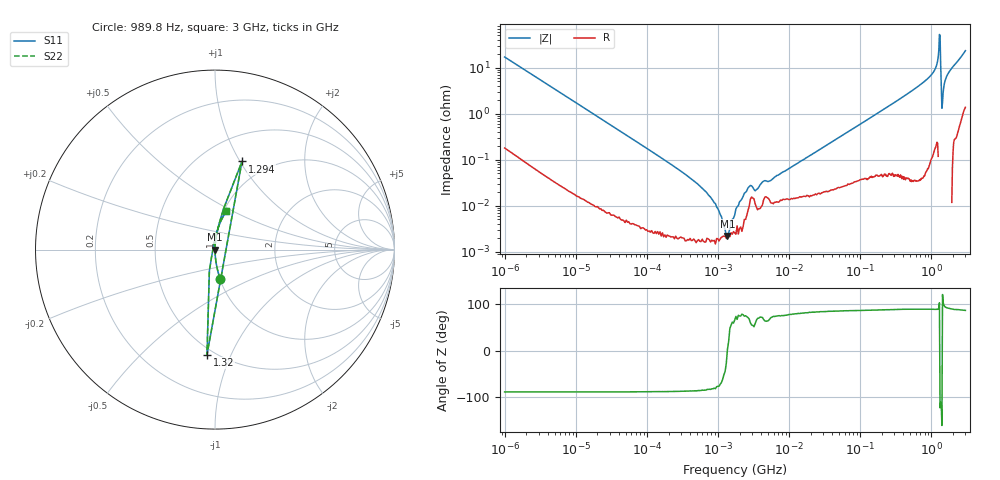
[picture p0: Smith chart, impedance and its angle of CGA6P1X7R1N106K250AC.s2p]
! S-Parameter Data Generated by TDK Corporation
! Copyright(C) 2020 TDK Corporation.
! All Rights Reserved.
! TDK P/N: CGA6P1X7R1N106K250AC (Multilayer Ceramic Chip Capacitor)
! Property: C=10uF
! Size(LxWxT): 3.2x2.5x2.5mm
! Model Type: s2p (Touchstone File Format Version 1.0)
! Frequency: DC=Yes Start=0.000989846MHz Stop=3000MHz 463points Log-sweep
! Model Generated on Aug. 18, 2020
! Port Assignments:
!  1 ---| |--- 2
! Applicable Conditions:
!  Temperature = 25 degC
!  DC Bias Voltage = 0 V
!  Small Signal Operation
! Terms and conditions regarding TDK Simulation Models
! (1)This simulation model is being provided solely for informational purposes. Please refer to the specifications of the products in terms of detailed characteristics of such products.
! (2)In no event shall TDK Corporation of any of its subsidiaries be liable for any loss or damage arising, directly or indirectly,
!  From any information contained in this simulation model, including, but not limited to loss or damages arising from any inaccuracies, omissions or errors in connection with such information.
! (3)Any and all copyrights on this simulation model are owned by TDK Corporation.
!  Duplication or redistribution of this simulation model without prior written permission from TDK Corporation is prohibited.
! (4)This simulation model is subject to any modification or change without any prior notice.
! (5)Neither TDK Corporation nor any of its subsidiaries shall make any warranty, express or implied,
!  Including but not limited to the correctness, implied warranties of merchantability and fitness for a particular purpose with respect to this simulation models.
! (6)The use of this simulation model shall be deemed to have consented to the terms and conditions hereof.
# Hz S MA R 50
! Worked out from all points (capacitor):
!   462 points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, 989.8 Hz to 3 GHz, reference 50 ohm
!   read as one part in series: C = 9.44 uF near 1.07 kHz
!   lowest |Z| = 2.18 mohm at 1.35 MHz (marker M1)
!   series resonance near 1.345 MHz, so ESL is about 1.5 nH
!   S11 on the Smith chart (normalised r, x): 989.8 Hz: 1.00, -0.34; 1.294 GHz: 0.76, +1.02; 1.32 GHz: 0.46, -0.82; 3 GHz: 1.03, +0.46
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989.846  0.167 -79.8  0.9842 9.6  0.9842 9.6  0.167 -79.8
12024.64  0.01431 -88.6  0.9998 0.8  0.9998 0.8  0.01431 -88.6
146075.1  0.001185 -88.8  1 0.1  1 0.1  0.001185 -88.8
489646.8  0.0003117 -87.1  1 0.0  1 0.0  0.0003117 -87.1
950504.9  9.329e-05 -78.1  1 0.0  1 0.0  9.329e-05 -78.1
1350401  2.178e-05 3.0  1 -0.0  1 -0.0  2.178e-05 3.0
1774518  8.504e-05 73.6  1 -0.0  1 -0.0  8.504e-05 73.6
2725710  0.0002585 68.2  0.9999 -0.0  0.9999 -0.0  0.0002585 68.2
3444703  0.0002229 65.4  0.9999 -0.0  0.9999 -0.0  0.0002229 65.4
2.073191e7  0.001291 82.7  0.9998 -0.1  0.9998 -0.1  0.001291 82.7
2.507343e8  0.01452 87.2  0.9994 -0.8  0.9994 -0.8  0.01452 87.2
9.779672e8  0.06695 85.3  0.9968 -3.8  0.9968 -3.8  0.06695 85.3
1.171007e9  0.1071 82.7  0.9921 -6.1  0.9921 -6.1  0.1071 82.7
1.243477e9  0.1662 80.0  0.9849 -9.6  0.9849 -9.6  0.1662 80.0
1.268618e9  0.2325 78.1  0.979 -13.4  0.979 -13.4  0.2325 78.1
1.294266e9  0.5134 73.0  0.9814 -30.0  0.9814 -30.0  0.5134 73.0
1.320433e9  0.5877 -94.4  1.198 29.3  1.198 29.3  0.5877 -94.4
1.374365e9  0.04248 -116.1  1.019 2.1  1.019 2.1  0.04248 -116.1
1.402151e9  0.0132 -161.5  1.013 0.2  1.013 0.2  0.0132 -161.5
1.430499e9  0.01749 120.0  1.009 -0.9  1.009 -0.9  0.01749 120.0
1.67892e9  0.06998 87.9  0.9998 -4.0  0.9998 -4.0  0.06998 87.9
3e9  0.2238 73.7  0.9616 -12.9  0.9616 -12.9  0.2238 73.7
